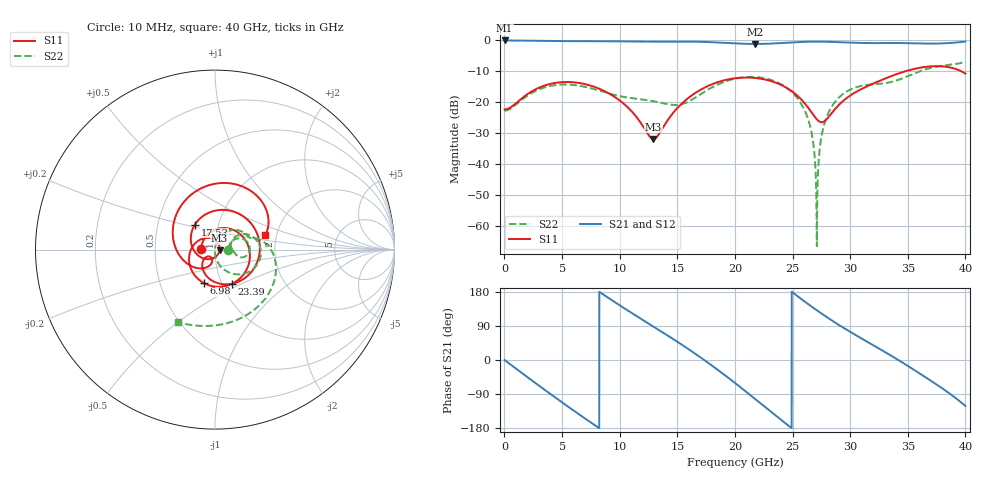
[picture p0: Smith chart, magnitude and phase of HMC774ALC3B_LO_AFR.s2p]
! Analog Devices, Inc.
! 1 Analog Way
! Wilmington, MA 01887
! http://www.analog.com
! Date:  2021-09-17 NN
! Board Name:  EV1HMC774ALC3B Revision A with HMC774ALC3B installed
! File Description:  Automatic Fixture Removal S-Parameters for LO Port connector and board loss de-embedding
! File Generation:  Calibrated Network Analyzer
! Chip Part Number:  HMC774ALC3B
! Chip Description:  MMIC, Double Balanced Mixer
! Chip Frequency:  7 to 34 GHz
! Chip Package:  LCC, 2.9 x 2.9 x 0.8 mm
! LO Port:  HMC774ALC3B removed and end of trace left open
! Note:
!  Analog Devices supplies this data as a sample of measured data at the evaluation board
!  ports for this product.  Your particular data for this product may vary.
!  Analog Devices reserves the right to change this data at anytime.
!  All lines below in this file are as is from the Network Analyzer.
!Agilent Technologies,N5245A,MY52451809,A.10.47.06
!Automatic Fixture Removal (AFR)
!Date: Friday, September 17, 2021 5:44:56 AM
!S2P File: Measurements: S11,S21,S12,S22:
# MHz S  RI  R 50
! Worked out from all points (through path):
!   4000 points, 10 MHz to 40 GHz, reference 50 ohm
!   highest |S21| = 0.00 dB at 10 MHz (marker M1); lowest = -1.1 dB at 21.78 GHz (marker M2)
!   group delay of S21, straight-line fit = 58.5 ps
!   lowest |S11| = -31.9 dB at 12.93 GHz (marker M3), VSWR 1.05, Z = 52.6 - j0.41 ohm
!   |S11| at or under -10 dB: start of sweep to 34.77 GHz; 39.66 GHz to end of sweep
!   |S22| runs from -66.5 to -6.9 dB; largest |S21 - S12| = 1.5e-15
!   S11 on the Smith chart (normalised r, x): 10 MHz: 0.86, +0.00; 6.98 GHz: 0.83, -0.32; 17.53 GHz: 0.77, +0.22; 23.39 GHz: 1.11, -0.44; 40 GHz: 1.74, +0.30
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10  -0.0766 0.00102  0.9995 -0.00398  0.9995 -0.00398  0.0732 0.000386
3450  0.1846 0.022  0.2055 -0.9591  0.2055 -0.9591  0.1643 0.0551
6680  -0.0304 -0.1999  -0.8248 -0.5186  -0.8248 -0.5186  0.1802 -0.0289
6980  -0.0614 -0.1869  -0.8768 -0.4245  -0.8768 -0.4245  0.1746 -0.034
9520  -0.1215 0.0218  -0.8675 0.4279  -0.8675 0.4279  0.1266 -0.0368
12930  0.0252 -0.0039  0.0314 0.955  0.0314 0.955  0.1033 -0.0114
13340  0.0186 -0.0227  0.1604 0.9424  0.1604 0.9424  0.1 -0.0079
15730  -0.1067 -0.02  0.7992 0.5299  0.7992 0.5299  0.0903 0.0377
17530  -0.1114 0.1398  0.9414 -0.071  0.9414 -0.071  0.1315 0.0814
20010  0.1699 0.1762  0.4387 -0.7814  0.4387 -0.7814  0.2362 0.0459
21780  0.2414 -0.0516  -0.2056 -0.8531  -0.2056 -0.8531  0.2498 -0.0531
23390  0.0936 -0.1906  -0.7153 -0.5364  -0.7153 -0.5364  0.1803 -0.1277
25550  -0.0702 -0.0988  -0.9116 0.2335  -0.9116 0.2335  0.0386 -0.1007
26670  -0.0522 -0.0435  -0.7377 0.6063  -0.7377 0.6063  0.00135 -0.0306
27120  -0.0368 -0.0377  -0.6258 0.723  -0.6258 0.723  -0.000279 0.00103
27640  -0.0218 -0.0427  -0.4765 0.8273  -0.4765 0.8273  0.00746 0.0359
28610  -0.0174 -0.0725  -0.1707 0.929  -0.1707 0.929  0.0441 0.0864
30750  -0.1223 -0.0962  0.4428 0.7985  0.4428 0.7985  0.149 0.1012
33340  -0.2354 0.0977  0.8766 0.2419  0.8766 0.2419  0.1978 0.0653
36290  0.00501 0.3677  0.6772 -0.5801  0.6772 -0.5801  0.327 -0.0319
38200  0.2455 0.287  0.1685 -0.8837  0.1685 -0.8837  0.2586 -0.2984
40000  0.2798 0.0796  -0.4982 -0.819  -0.4982 -0.819  -0.2077 -0.4038
